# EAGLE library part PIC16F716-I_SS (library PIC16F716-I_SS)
Microchip PIC16F716-I/SS, 8bit PIC16F Microcontroller, 20MHz, 3.5 kB Flash, 20-Pin SSOP Source: Datasheet
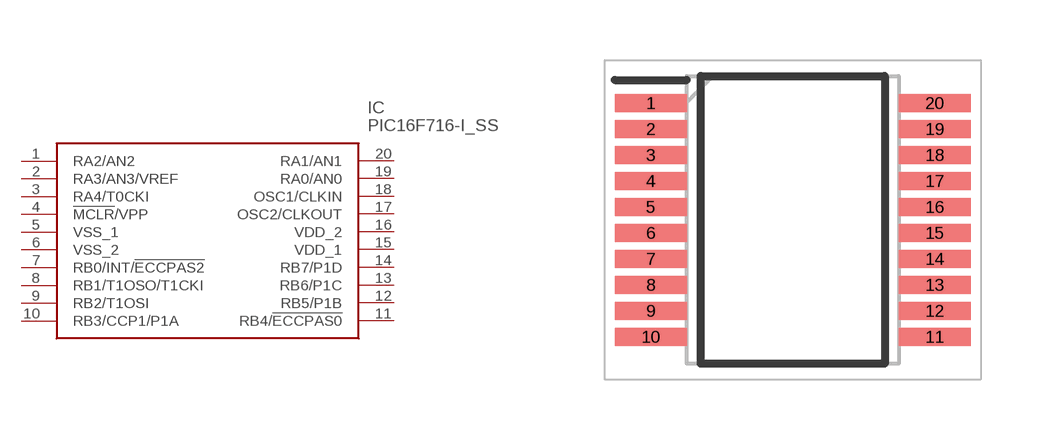
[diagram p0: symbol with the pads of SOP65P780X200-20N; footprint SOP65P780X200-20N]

Designator prefix IC

## PIC16F716-I_SS (Description: Microchip PIC16F716-I/SS, 8bit PIC16F Microcontroller, 20MHz, 3.5 kB Flash, 20-Pin SSOP; Height: 2mm; Manufacturer_Name: Microchip; Manufacturer_Part_Number: PIC16F716-I/SS; Mouser_Part_Number: 579-PIC16F716-I/SS; Mouser_Price-Stock: https://www.mouser.co.uk/ProductDetail/Microchip-Technology-Atmel/PIC16F716-I-SS?qs=z30FE1aq6wY%2Fe40zUIPEhw%3D%3D)  [SOP65P780X200-20N]
1  RA2/AN2
2  RA3/AN3/VREF
3  RA4/T0CKI
4  !MCLR!/VPP
5  VSS_1
6  VSS_2
7  RB0/INT/!ECCPAS2
8  RB1/T1OSO/T1CKI
9  RB2/T1OSI
10  RB3/CCP1/P1A
11  RB4/!ECCPAS0
12  RB5/P1B
13  RB6/P1C
14  RB7/P1D
15  VDD_1
16  VDD_2
17  OSC2/CLKOUT
18  OSC1/CLKIN
19  RA0/AN0
20  RA1/AN1

## Footprint SOP65P780X200-20N (pad centres in mm)
(SS)20-lead(SSOP)
smd 1.8 x 0.45: 1 -3.55,2.925; 2 -3.55,2.275; 3 -3.55,1.625; 4 -3.55,0.975; 5 -3.55,0.325; 6 -3.55,-0.325; 7 -3.55,-0.975; 8 -3.55,-1.625; 9 -3.55,-2.275; 10 -3.55,-2.925; 11 3.55,-2.925; 12 3.55,-2.275; 13 3.55,-1.625; 14 3.55,-0.975; 15 3.55,-0.325; 16 3.55,0.325; 17 3.55,0.975; 18 3.55,1.625; 19 3.55,2.275; 20 3.55,2.925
